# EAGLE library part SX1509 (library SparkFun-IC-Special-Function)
Semtech SX1509 The SX1509 is a complete ultra low voltage 1.2V to 3.6V General Purpose parallel Input/Output (GPIO) expanders ideal for low power handheld battery powered equipment. This version comes in a 16-channel configuration and allows easy serial expansion of I/O through a standard 400kHz I2C interface. GPIO devices can provide additional control and monitoring when the microcontroller or chipset has insufficient I/O ports, or in systems where serial communication and control from a remote location is advantageous. Datasheet SparkFun Products SparkFun 16 Output I/O Expander Breakout - SX1509 (BOB-13601) SparkFun Line Follower Array (SEN-13582)
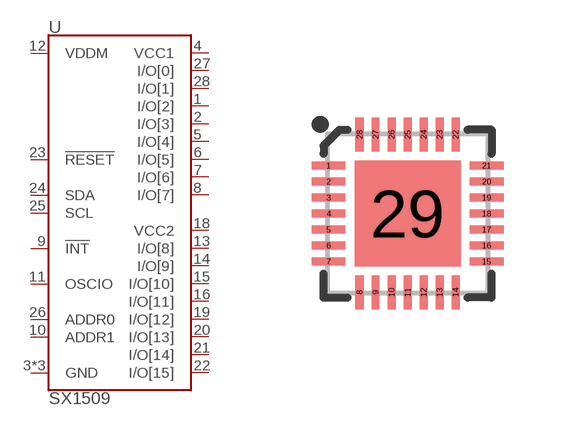
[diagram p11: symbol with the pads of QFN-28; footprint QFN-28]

Designator prefix U

## SX1509 (PROD_ID: IC-11311; VALUE: SX1509)  [QFN-28]
1  I/O[2]
2  I/O[3]
3  GND
4  VCC1
5  I/O[4]
6  I/O[5]
7  I/O[6]
8  I/O[7]
9  !INT
10  ADDR1
11  OSCIO
12  VDDM
13  I/O[8]
14  I/O[9]
15  I/O[10]
16  I/O[11]
17  GND
18  VCC2
19  I/O[12]
20  I/O[13]
21  I/O[14]
22  I/O[15]
23  !RESET
24  SDA
25  SCL
26  ADDR0
27  I/O[0]
28  I/O[1]
29  GND

## Footprint QFN-28 (pad centres in mm)
smd 0.85 x 0.2: 1 -1.975,1.2; 2 -1.975,0.8; 3 -1.975,0.4; 4 -1.975,0; 5 -1.975,-0.4; 6 -1.975,-0.8; 7 -1.975,-1.2; 15 1.975,-1.2; 16 1.975,-0.8; 17 1.975,-0.4; 18 1.975,0; 19 1.975,0.4; 20 1.975,0.8; 21 1.975,1.2
smd 0.2 x 0.85: 8 -1.2,-1.975; 9 -0.8,-1.975; 10 -0.4,-1.975; 11 0,-1.975; 12 0.4,-1.975; 13 0.8,-1.975; 14 1.2,-1.975; 22 1.2,1.975; 23 0.8,1.975; 24 0.4,1.975; 25 0,1.975; 26 -0.4,1.975; 27 -0.8,1.975; 28 -1.2,1.975
smd 2.65 x 2.65: 29 0,0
